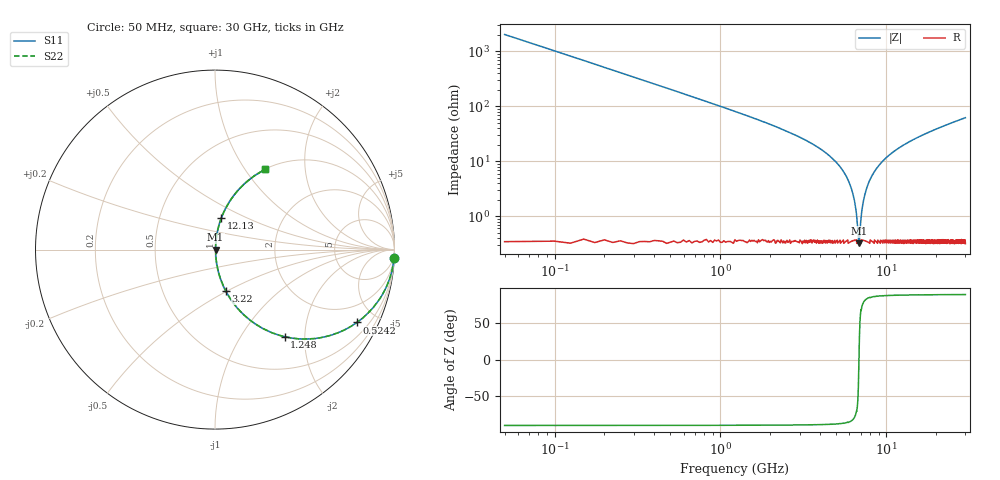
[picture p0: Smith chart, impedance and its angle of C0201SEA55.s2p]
!	AVX Thin Film Operation 	Date: April 2014
!	Description: Accu-P® Series, Thin Film  SMD RF Capacitor
!	Part Number: 02015JA55PBSTR
# MHZ S MA R 50
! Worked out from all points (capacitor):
!   1201 points, 50 MHz to 30 GHz, reference 50 ohm
!   read as one part in series: C = 1.55 pF near 199.8 MHz
!   lowest |Z| = 325 mohm at 6.839 GHz (marker M1)
!   series resonance near 6.845 GHz, so ESL is about 350 pH
!   S11 on the Smith chart (normalised r, x): 50 MHz: 1, -41; 524.2 MHz: 1.01, -3.89; 1.248 GHz: 1.01, -1.59; 3.22 GHz: 1.01, -0.50; 12.13 GHz: 1.01, +0.36; 30 GHz: 1.01, +1.25
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50  0.999 -2.8  0.049 87.2  0.049 87.2  0.999 -2.8
274.625  0.966 -15.0  0.259 75.0  0.259 75.0  0.966 -15.0
524.208  0.889 -27.2  0.456 62.7  0.456 62.7  0.889 -27.2
1248  0.621 -51.3  0.781 38.4  0.781 38.4  0.621 -51.3
2046.667  0.414 -65.1  0.907 24.5  0.907 24.5  0.414 -65.1
3219.708  0.24 -75.3  0.967 13.9  0.967 13.9  0.24 -75.3
5041.667  0.093 -82.6  0.992 5.3  0.992 5.3  0.093 -82.6
5690.583  0.056 -83.3  0.995 3.2  0.995 3.2  0.056 -83.3
6164.792  0.032 -81.9  0.996 1.8  0.996 1.8  0.032 -81.9
6464.292  0.017 -77.6  0.996 1.0  0.996 1.0  0.017 -77.6
6738.833  0.005813 -53.2  0.997 0.3  0.997 0.3  0.005813 -53.2
6838.667  0.003469 -4.5  0.997 0.0  0.997 0.0  0.003469 -4.5
6938.5  0.005331 49.3  0.997 -0.2  0.997 -0.2  0.005331 49.3
7287.917  0.019 78.5  0.996 -1.1  0.996 -1.1  0.019 78.5
7787.083  0.039 82.7  0.996 -2.2  0.996 -2.2  0.039 82.7
8760.458  0.074 83.1  0.994 -4.3  0.994 -4.3  0.074 83.1
10058.29  0.117 81.6  0.99 -6.7  0.99 -6.7  0.117 81.6
12129.83  0.178 78.7  0.981 -10.2  0.981 -10.2  0.178 78.7
15025  0.252 74.7  0.964 -14.6  0.964 -14.6  0.252 74.7
20016.67  0.36 68.4  0.93 -21.1  0.93 -21.1  0.36 68.4
25033.29  0.451 62.8  0.889 -26.8  0.889 -26.8  0.451 62.8
30000  0.528 57.8  0.847 -31.8  0.847 -31.8  0.528 57.8
